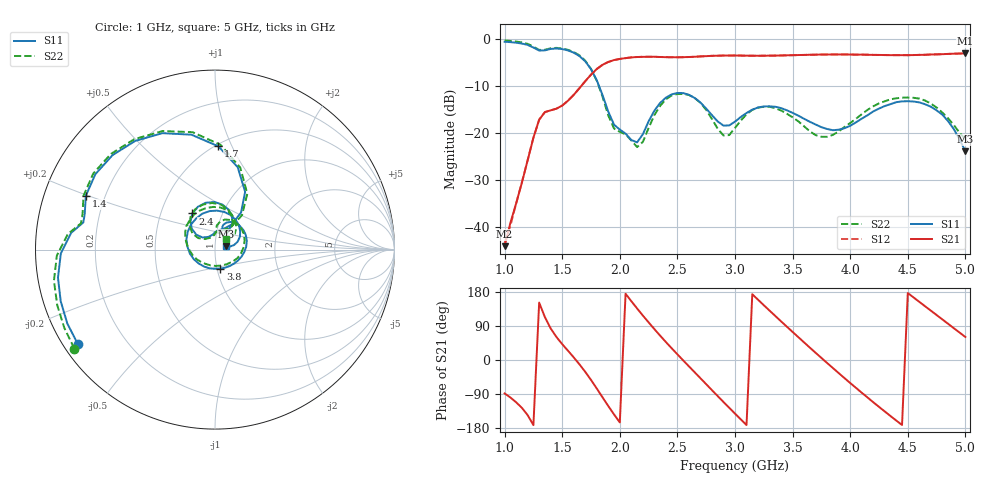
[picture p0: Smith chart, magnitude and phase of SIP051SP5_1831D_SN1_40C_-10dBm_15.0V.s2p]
# GHz  S  dB  R  50
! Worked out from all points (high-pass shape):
!   81 points, 1 GHz to 5 GHz, reference 50 ohm
!   highest |S21| = -3.12 dB at 5 GHz (marker M1); lowest = -44.0 dB at 1 GHz (marker M2)
!   |S21| within 3 dB of the highest: 1.817 GHz to end of sweep
!   lowest |S11| = -23.9 dB at 5 GHz (marker M3), VSWR 1.14, Z = 56.5 + j2.15 ohm
!   |S11| at or under -10 dB: 1.819 GHz to end of sweep
!   |S22| runs from -23.0 to -0.4 dB; largest |S21 - S12| = 0.002
!   S11 on the Smith chart (normalised r, x): 1 GHz: 0.04, -0.31; 1.4 GHz: 0.13, +0.20; 1.7 GHz: 0.52, +0.89; 2.4 GHz: 0.72, +0.31; 3.8 GHz: 1.04, -0.22; 5 GHz: 1.13, +0.04
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1  -0.65 -145.6  -43.99 -88.2  -43.28 -89.7  -0.37 -144.8
1.3  -2.51 168.3  -17.17 151.4  -17.18 151.4  -2.37 168.9
1.4  -2.16 157.4  -15.19 83.2  -15.18 83.2  -2.03 157.7
1.55  -2.48 126.2  -13.15 24.5  -13.16 24.5  -2.36 126.2
1.7  -4.79 88.1  -9.00 -31.3  -9.02 -31.3  -4.67 86.9
1.85  -11.95 54.9  -5.53 -98.5  -5.53 -98.4  -12.29 51.8
2.05  -20.12 88.5  -4.12 174.9  -4.12 174.8  -20.28 87.0
2.2  -20.26 135.8  -3.84 117.4  -3.84 117.4  -21.89 133.2
2.35  -13.61 131.0  -3.88 64.3  -3.87 64.3  -14.24 136.8
2.4  -12.50 122.0  -3.92 47.4  -3.91 47.4  -12.86 126.9
2.55  -11.53 90.7  -3.92 -0.9  -3.92 -0.9  -11.69 93.5
2.75  -14.82 57.5  -3.70 -63.9  -3.69 -63.9  -15.09 55.8
3  -17.58 72.2  -3.56 -141.5  -3.56 -141.5  -18.92 86.4
3.2  -14.58 52.7  -3.62 159.0  -3.62 159.1  -14.61 62.6
3.4  -14.71 15.3  -3.56 101.9  -3.55 102.0  -15.22 17.9
3.7  -18.19 -48.0  -3.39 18.9  -3.38 19.0  -20.44 -69.4
3.8  -19.14 -74.6  -3.36 -8.0  -3.35 -8.0  -20.80 -106.1
4.1  -16.95 -171.2  -3.37 -86.3  -3.37 -86.3  -16.01 170.2
4.35  -13.87 121.6  -3.49 -147.9  -3.49 -147.9  -12.85 120.6
4.6  -13.50 65.4  -3.43 153.4  -3.43 153.4  -12.70 74.3
4.8  -16.10 27.4  -3.28 107.0  -3.27 107.1  -15.66 44.5
5  -23.86 17.2  -3.12 60.7  -3.12 60.8  -21.33 42.8
